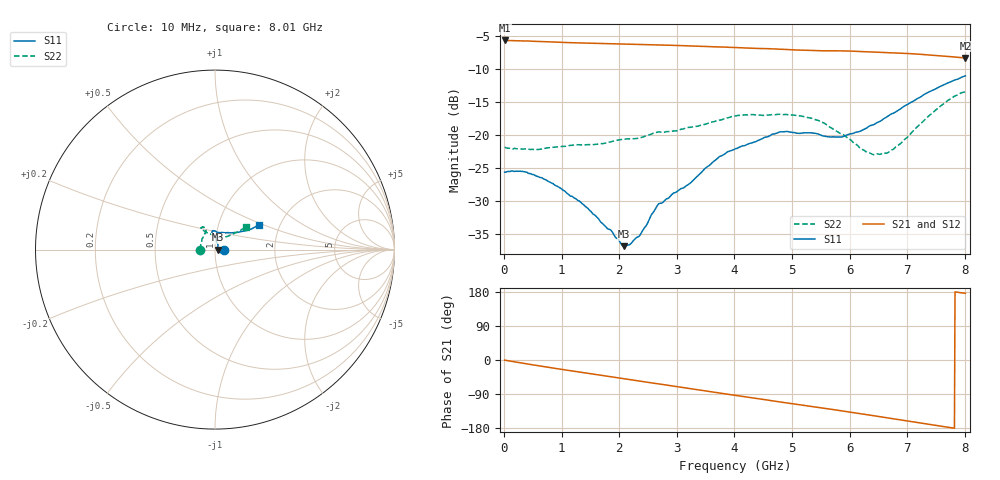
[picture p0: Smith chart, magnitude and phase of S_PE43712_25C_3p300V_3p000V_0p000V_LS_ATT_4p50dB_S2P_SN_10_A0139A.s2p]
! DEVICE ID: PE43712
! File Path: z:\PE43713\PE43713_CHAR_NOM_04292014\AMB\3p300\LS_ATT_4p50dB\PE43713_AMB_3p300V_3p000V_0p000V_LS_ATT_4p50dB_S2P_SN_10_A0139A.s2p
! Serial: 10
! Lot: A0139A
! Temp: 25C
! VDD: 3.300
! VSS: 0.000
! Control_Hi: 3.000
! Control_Lo: 0.000
! Attenuation Step: 4.50dB
! Port 1: RF1
! Port 2: RF2
! ThroughPath:1-2
! IDD: 0.0001467274
! ISS: -3.24e-008
#  Hz  S  RI  R  50
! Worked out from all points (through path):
!   801 points, 10 MHz to 8.01 GHz, reference 50 ohm
!   highest |S21| = -5.60 dB at 10 MHz (marker M1); lowest = -8.3 dB at 8.01 GHz (marker M2)
!   group delay of S21, straight-line fit = 63.1 ps
!   lowest |S11| = -36.8 dB at 2.08 GHz (marker M3), VSWR 1.03, Z = 51.5 - j0.0174 ohm
!   |S11| at or under -10 dB: start of sweep to end of sweep
!   |S22| runs from -22.9 to -13.4 dB; largest |S21 - S12| = 0.0016
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1e7  0.0526 -0.000103  0.5245 -0.00302  0.5243 -0.00278  -0.0812 0.000465
3.4e8  0.0521 -0.0102  0.5134 -0.0798  0.5131 -0.0786  -0.0785 0.00634
6.3e8  0.0455 -0.0153  0.495 -0.1414  0.4949 -0.1414  -0.0776 0.0127
9.6e8  0.0363 -0.0174  0.4652 -0.2053  0.4653 -0.2053  -0.0794 0.0209
1.35e9  0.0262 -0.0156  0.4223 -0.2713  0.4222 -0.2713  -0.0788 0.0317
1.86e9  0.0183 -0.00515  0.3544 -0.3458  0.3544 -0.3457  -0.0734 0.0512
2.08e9  0.0145 -0.000169  0.3211 -0.3735  0.3211 -0.3733  -0.0727 0.0588
2.18e9  0.0146 0.00285  0.3053 -0.3851  0.3054 -0.3849  -0.0706 0.0623
2.36e9  0.0143 0.0101  0.2751 -0.4042  0.2751 -0.404  -0.0647 0.0707
2.68e9  0.017 0.0249  0.2204 -0.4307  0.2204 -0.4307  -0.0546 0.0914
3.22e9  0.00898 0.0421  0.1207 -0.4614  0.1208 -0.4615  -0.0522 0.1025
3.72e9  0.00331 0.0678  0.028 -0.4678  0.0279 -0.4677  -0.0548 0.1177
4.01e9  -0.00401 0.0789  -0.0258 -0.4633  -0.0257 -0.4633  -0.0644 0.1248
4.79e9  -0.0146 0.1054  -0.1583 -0.4214  -0.1583 -0.4217  -0.077 0.1224
5.35e9  -0.00264 0.1042  -0.2386 -0.3704  -0.2385 -0.3701  -0.0746 0.112
5.86e9  0.0248 0.094  -0.3044 -0.3137  -0.304 -0.3137  -0.041 0.0936
6.34e9  0.0694 0.0949  -0.3531 -0.2451  -0.3524 -0.2449  0.000526 0.0738
6.68e9  0.105 0.0946  -0.378 -0.1906  -0.3777 -0.1907  0.0329 0.0671
6.88e9  0.1264 0.0957  -0.3895 -0.1576  -0.3891 -0.1575  0.052 0.069
7.56e9  0.2029 0.1159  -0.3989 -0.0409  -0.3986 -0.0411  0.1297 0.1013
7.81e9  0.2271 0.1293  -0.3934 -0.00176  -0.3932 -0.00198  0.1581 0.1179
8.01e9  0.2462 0.1392  -0.3854 0.0266  -0.3848 0.026  0.1725 0.127
